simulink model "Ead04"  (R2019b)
settings: Solver=FixedStepDiscrete  StartTime=0.0  StopTime=20  FixedStep=1  RelTol=1e-3

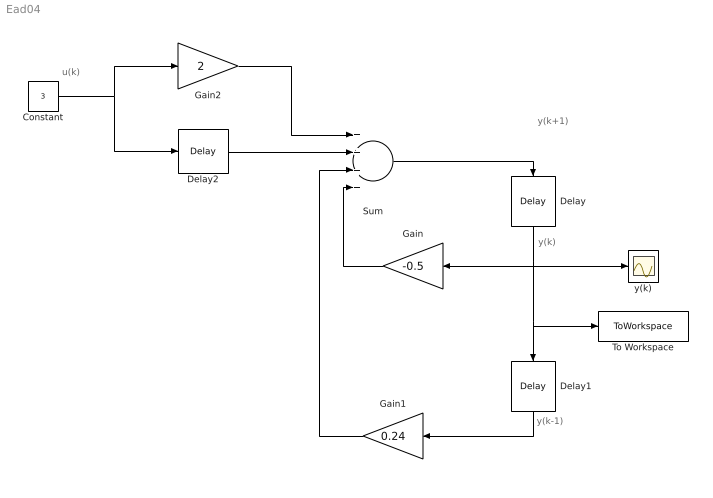
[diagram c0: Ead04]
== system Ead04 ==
  note: y(k+1)
  note: y(k)
  note: y(k-1)
  note: u(k)
  Constant : Constant  Value=3
  Delay : Delay  DelayLength=1  InitialCondition=2
  Delay1 : Delay  DelayLength=1  InitialCondition=20.83
  Delay2 : Delay  DelayLength=1  InitialCondition=0
  Gain : Gain  Gain=-0.5
  Gain1 : Gain  Gain=0.24
  Gain2 : Gain  Gain=2
  Sum : Sum  Inputs=++++
  To Workspace : ToWorkspace  VariableName=y  SaveFormat=Timeseries  SampleTime=-1
  y(k) : Scope
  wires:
  Delay/1 -> y(k)/1, To Workspace/1, Delay1/1, Gain/1
  Sum/1 -> Delay/1
  Delay1/1 -> Gain1/1
  Constant/1 -> Gain2/1, Delay2/1
  Gain2/1 -> Sum/1
  Delay2/1 -> Sum/2
  Gain/1 -> Sum/4
  Gain1/1 -> Sum/3
